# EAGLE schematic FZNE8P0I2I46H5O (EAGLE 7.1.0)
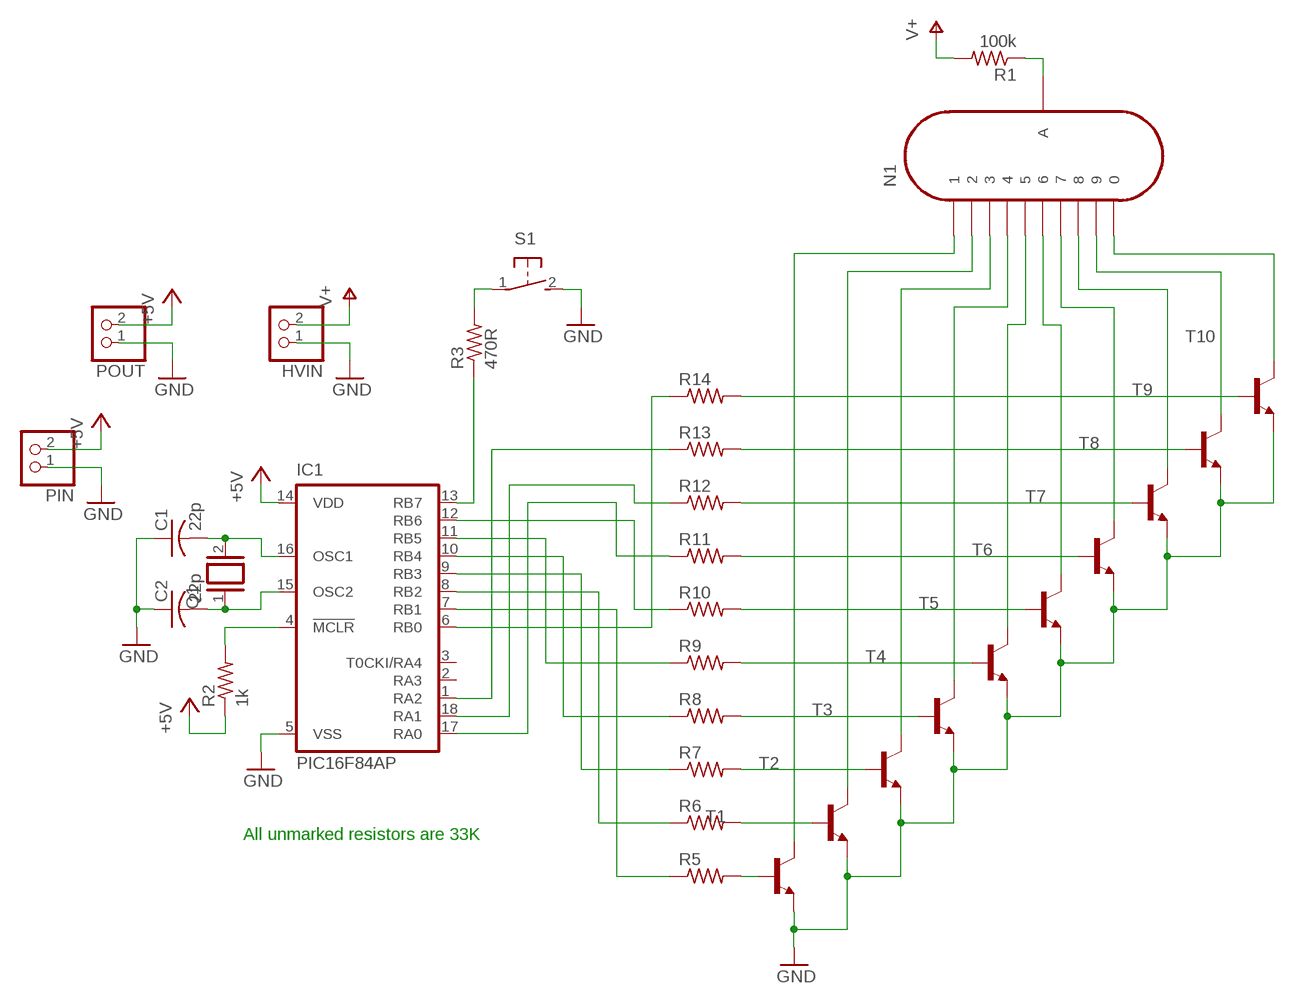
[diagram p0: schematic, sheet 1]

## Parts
C1  22p  C-USC0805  [C0805]
C2  22p  C-USC0805  [C0805]
HVIN  PINHD-1X2  [1X02]
IC1  PIC16F84AP  [DIL18]
N1  IN-12A  [IN-12]
PIN  PINHD-1X2/90  [1X02/90]
POUT  PINHD-1X2  [1X02]
Q1  XTAL/S  [QS]
R1  100k  R-US_R0805  [R0805]
R2  1k  R-US_R0805  [R0805]
R3  470R  R-US_R0805  [R0805]
R5  R-US_R0805  [R0805]
R6  R-US_R0805  [R0805]
R7  R-US_R0805  [R0805]
R8  R-US_R0805  [R0805]
R9  R-US_R0805  [R0805]
R10  R-US_R0805  [R0805]
R11  R-US_R0805  [R0805]
R12  R-US_R0805  [R0805]
R13  R-US_R0805  [R0805]
R14  R-US_R0805  [R0805]
S1  31-XX  [B3F-31XX]
T1  MMBTA42LT1-NPN-SOT23-BEC  [SOT23-BEC]
T2  MMBTA42LT1-NPN-SOT23-BEC  [SOT23-BEC]
T3  MMBTA42LT1-NPN-SOT23-BEC  [SOT23-BEC]
T4  MMBTA42LT1-NPN-SOT23-BEC  [SOT23-BEC]
T5  MMBTA42LT1-NPN-SOT23-BEC  [SOT23-BEC]
T6  MMBTA42LT1-NPN-SOT23-BEC  [SOT23-BEC]
T7  MMBTA42LT1-NPN-SOT23-BEC  [SOT23-BEC]
T8  MMBTA42LT1-NPN-SOT23-BEC  [SOT23-BEC]
T9  MMBTA42LT1-NPN-SOT23-BEC  [SOT23-BEC]
T10  MMBTA42LT1-NPN-SOT23-BEC  [SOT23-BEC]

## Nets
+5V: IC1.14(VDD) PIN.2 POUT.2 R2.1
GND: C1.1 C2.1 HVIN.1 IC1.5(VSS) PIN.1 POUT.1 S1.2(S) T1.E T2.E T3.E T4.E T5.E T6.E T7.E T8.E T9.E T10.E
N$1: N1.0 T10.C
N$2: N1.9 T9.C
N$3: N1.8 T8.C
N$4: N1.7 T7.C
N$5: N1.6 T6.C
N$6: N1.5 T5.C
N$7: N1.1 T1.C
N$8: N1.2 T2.C
N$9: N1.3 T3.C
N$10: N1.4 T4.C
N$11: C1.2 IC1.16(OSC1) Q1.2
N$12: IC1.4(!MCLR) R2.2
N$13: C2.2 IC1.15(OSC2) Q1.1
N$14: IC1.13(RB7) R3.1
N$15: R3.2 S1.1(P)
N$16: IC1.6(RB0) R14.1
N$17: IC1.7(RB1) R5.1
N$18: R5.2 T1.B
N$19: R6.2 T2.B
N$20: R7.2 T3.B
N$21: IC1.8(RB2) R6.1
N$22: N1.A R1.1
N$23: IC1.9(RB3) R7.1
N$24: IC1.10(RB4) R8.1
N$25: IC1.11(RB5) R9.1
N$26: IC1.12(RB6) R10.1
N$27: IC1.17(RA0) R11.1
N$28: IC1.18(RA1) R12.1
N$29: IC1.1(RA2) R13.1
N$32: R8.2 T4.B
N$33: R9.2 T5.B
N$34: R10.2 T6.B
N$35: R11.2 T7.B
N$36: R12.2 T8.B
N$37: R13.2 T9.B
N$38: R14.2 T10.B
V+: HVIN.2 R1.2
Unconnected: IC1.2(RA3) IC1.3(T0CKI/RA4)

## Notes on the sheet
- All unmarked resistors are 33K

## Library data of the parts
C1 C2 = rcl:C-US: CAPACITOR, American symbol
HVIN PIN POUT = pinhead:PINHD-1X2: PIN HEADER
IC1 = microchip:PIC16F8*: MICROCONTROLLER 8-Bit PIC16F8X Family - CMOS Flash/EEPROM Pin Compatible : PIC16F83, PIC16CR83, PIC16F84A, PIC16CR84 see also PIC16C*; MF: MICROCHIP; MPN: PIC16F84A-04I/P; OC_FARNELL: 9760865; OC_NEWARK: 69K7635
N1 = russian-nixies:IN-12A: IN-12A: medium numeric topview nixie tube
Q1 = special:XTAL/S: CRYSTAL
R1-R3 R5-R14 = rcl:R-US_: RESISTOR, American symbol
S1 = switch-omron:31-XX: OMRON SWITCH; MPN: B3F-3100; OC_FARNELL: 959704; OC_NEWARK: 36M3582
T1-T10 = transistor:*-NPN-: NPN Transistror BF959 corrected 2008.03.06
